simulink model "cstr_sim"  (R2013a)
settings: Solver=ode45  StartTime=0.0  StopTime=20  RelTol=1e-3

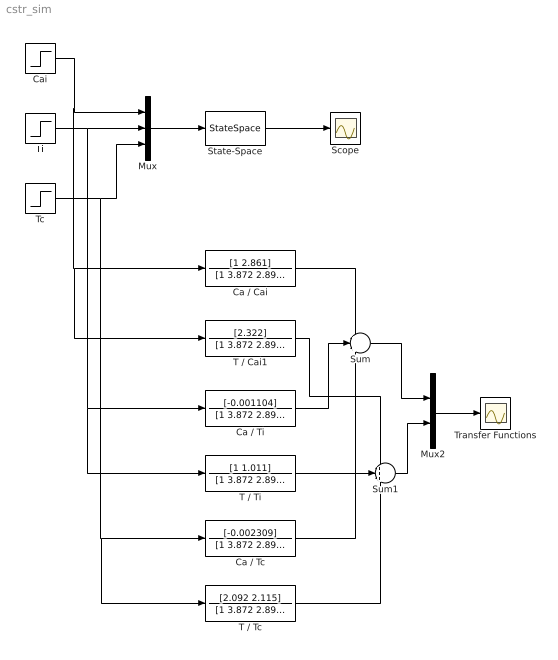
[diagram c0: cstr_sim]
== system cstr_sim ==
  Ca / Cai : TransferFcn  Numerator=[1 2.861]  Denominator=[1 3.872 2.895]
  Ca / Tc : TransferFcn  Numerator=[-0.002309]  Denominator=[1 3.872 2.895]
  Ca / Ti : TransferFcn  Numerator=[-0.001104]  Denominator=[1 3.872 2.895]
  Cai : Step  SampleTime=0
  Mux : Mux  Inputs=3
  Mux2 : Mux  Inputs=2
  Scope : Scope
  State-Space : StateSpace  A="[-1.011  -0.001104; 2.322     -2.861]"  B="[1 0 0; 0 1  2.092]"  C=[1 0; 0 1]  D=[0 0 0; 0 0 0]
  Sum : Sum  Inputs=+++
  Sum1 : Sum  Inputs=+++
  T / Cai1 : TransferFcn  Numerator=[2.322]  Denominator=[1 3.872 2.895]
  T / Tc : TransferFcn  Numerator=[2.092 2.115]  Denominator=[1 3.872 2.895]
  T / Ti : TransferFcn  Numerator=[1 1.011]  Denominator=[1 3.872 2.895]
  Tc : Step  Time=10  SampleTime=0
  Ti : Step  Time=5  SampleTime=0
  Transfer Functions : Scope
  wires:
  Cai/1 -> Mux/1, T / Cai1/1, Ca / Cai/1
  Ti/1 -> T / Ti/1, Ca / Ti/1, Mux/2
  Tc/1 -> T / Tc/1, Ca / Tc/1, Mux/3
  Mux/1 -> State-Space/1
  State-Space/1 -> Scope/1
  Ca / Cai/1 -> Sum/1
  Ca / Ti/1 -> Sum/2
  Ca / Tc/1 -> Sum/3
  T / Cai1/1 -> Sum1/1
  T / Ti/1 -> Sum1/2
  T / Tc/1 -> Sum1/3
  Sum1/1 -> Mux2/2
  Sum/1 -> Mux2/1
  Mux2/1 -> Transfer Functions/1
